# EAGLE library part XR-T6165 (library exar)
Codirectional digital PROCESSOR
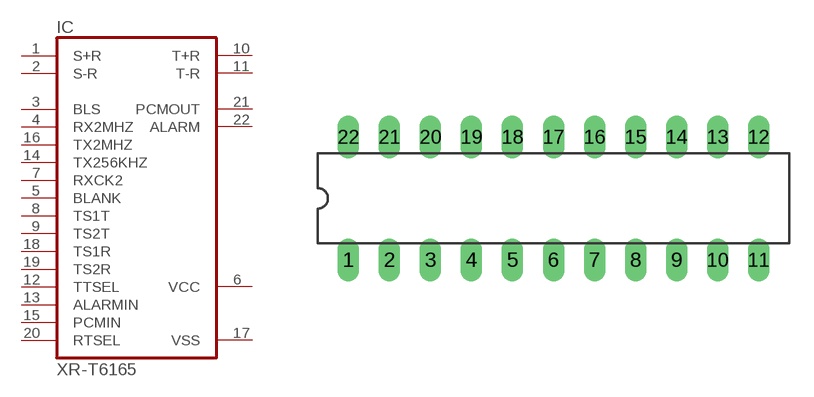
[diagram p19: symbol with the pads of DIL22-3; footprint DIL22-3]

Designator prefix IC

## XR-T6165 (OC_FARNELL: unknown; OC_NEWARK: unknown)  [DIL22-3]
1  S+R  in
2  S-R  in
3  BLS  in
4  RX2MHZ  in
5  BLANK  in
6  VCC  pwr
7  RXCK2  in
8  TS1T  in
9  TS2T  in
10  T+R  out
11  T-R  out
12  TTSEL  in
13  ALARMIN  in
14  TX256KHZ  in
15  PCMIN  in
16  TX2MHZ  in
17  VSS  pwr
18  TS1R  in
19  TS2R  in
20  RTSEL  in
21  PCMOUT  out
22  ALARM  out

## Footprint DIL22-3 (pad centres in mm)
Dual In Line Package 0.3 inch
drill 0.813 long: 1 -12.7,-3.81; 2 -10.16,-3.81; 3 -7.62,-3.81; 4 -5.08,-3.81; 5 -2.54,-3.81; 6 0,-3.81; 7 2.54,-3.81; 8 5.08,-3.81; 9 7.62,-3.81; 10 10.16,-3.81; 11 12.7,-3.81; 12 12.7,3.81; 13 10.16,3.81; 14 7.62,3.81; 15 5.08,3.81; 16 2.54,3.81; 17 0,3.81; 18 -2.54,3.81; 19 -5.08,3.81; 20 -7.62,3.81; 21 -10.16,3.81; 22 -12.7,3.81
